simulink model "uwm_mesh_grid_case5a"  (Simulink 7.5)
settings: Solver=ode45  StartTime=0.0  StopTime=3.0  RelTol=1e-4
undefined symbols (not defined in the file or in its folder): D1, Delta, dfilt, DiscIntNeverNeededParam, Discrete, no, powergui, steady, ZData
libraries: powerlib x259, powerlib_extras x68, dsparch4 x11
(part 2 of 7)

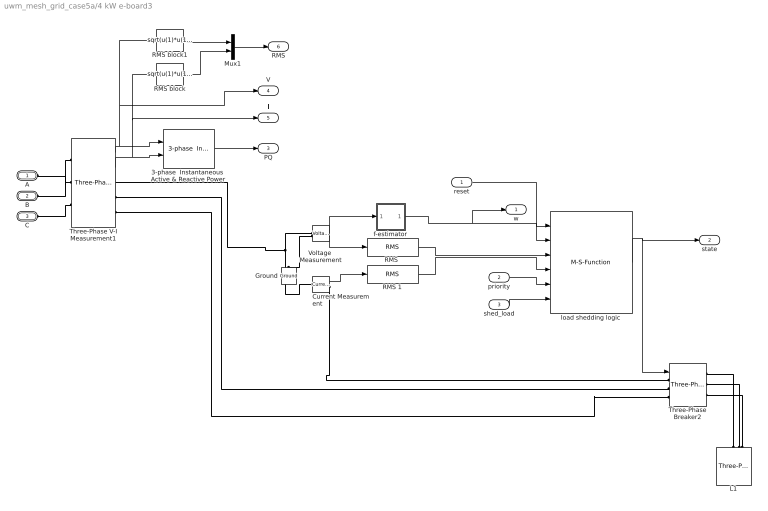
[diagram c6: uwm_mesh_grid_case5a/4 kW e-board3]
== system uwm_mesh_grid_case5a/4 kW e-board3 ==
  reset : Inport
  priority : Inport  Port=2
  shed_load : Inport  Port=3
  3-phase  Instantaneous  Active & Reactive Power : powerlib_extras/Measurements/3-phase  Instantaneous  Active & Reactive Power  DialogController=POWERSYS.PowerSysDialog  SystemSampleTime=-1
  Current Measurement : powerlib/Measurements/Current Measurement  DialogController=POWERSYS.PowerSysDialog  SystemSampleTime=-1  PhasorSimulation=off  OutputType=Complex  PSBequivalent=0
  Ground : powerlib/Elements/Ground  DialogController=POWERSYS.PowerSysDialog  PhysicalDomain=powersysdomain  SubClassName=unknown  LeftPortType=p1  RightPortType=p1  LConnTagsString=a
  L1 : powerlib/Elements/Three-Phase Series RLC Load  DialogController=POWERSYS.PowerSysDialog  PhysicalDomain=powersysdomain  SubClassName=unknown  LeftPortType=p1  RightPortType=p1  LConnTagsString=A|B|C  Configuration=Y (grounded)  NominalVoltage=208  NominalFrequency=60  ActivePower=4000  InductivePower=0  CapacitivePower=0  Measurements=None
  Mux1 : Mux  Inputs=2
  "RMS " : powerlib_extras/Measurements/RMS  DialogController=POWERSYS.PowerSysDialog  SystemSampleTime=-1  f1=60
  RMS 1 : powerlib_extras/Measurements/RMS  DialogController=POWERSYS.PowerSysDialog  SystemSampleTime=-1  f1=60
  RMS block : Fcn  Expr=sqrt(u(1)*u(1)+u(2)*u(2)+u(3)*u(3))/sqrt(3)
  RMS block1 : Fcn  Expr=sqrt(u(1)*u(1)+u(2)*u(2)+u(3)*u(3))/sqrt(3)
  Three-Phase V-I Measurement1 : powerlib/Measurements/Three-Phase V-I Measurement  DialogController=POWERSYS.PowerSysDialog  SystemSampleTime=-1  VoltageMeasurement=phase-to-ground  SetLabelV=off  LabelV=Vabc  Vpu=off  VpuLL=off  CurrentMeasurement=yes  SetLabelI=off  LabelI=Iabc  Ipu=off  Pbase=100e6  Vbase=500e3  OutputType=Complex  PhasorSimulation=off  PSBequivalent=0
  Three-Phase Breaker2 : powerlib/Elements/Three-Phase Breaker  DialogController=POWERSYS.PowerSysDialog  SystemSampleTime=-1  InitialState=closed  SwitchA=on  SwitchB=on  SwitchC=on  SwitchTimes=[50]  External=on  BreakerResistance=0.001  SnubberResistance=1e6  SnubberCapacitance=inf  Measurements=None
  Voltage  Measurement : powerlib/Measurements/Voltage Measurement  DialogController=POWERSYS.PowerSysDialog  SystemSampleTime=-1  PhasorSimulation=off  OutputType=Complex  PSBequivalent=0
  f-estimator : Subsystem  mask{dt=0.010}
      mask prompts: dt "sample time"
  load shedding logic : M-S-Function  FunctionName=load_shedding_logic3
  A : PMIOPort  Port=1  Side=Left
  B : PMIOPort  Port=2  Side=Left
  C : PMIOPort  Port=3  Side=Left
  w : Outport  OutDataType=fixdt(1, 16)  OutScaling=2^0
  state : Outport  Port=2  OutDataType=fixdt(1, 16)  OutScaling=2^0
  PQ : Outport  Port=3  OutDataType=fixdt(1, 16)  OutScaling=2^0
  V : Outport  Port=4  OutDataType=fixdt(1, 16)  OutScaling=2^0
  I : Outport  Port=5  OutDataType=fixdt(1, 16)  OutScaling=2^0
  RMS : Outport  Port=6  OutDataType=fixdt(1, 16)  OutScaling=2^0
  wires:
  reset/1 -> load shedding logic/1
  Current Measurement/1 -> RMS 1/1
  Voltage  Measurement/1 -> "RMS "/1, f-estimator/1(v)
  f-estimator/1(w) -> load shedding logic/2, w/1
  "RMS "/1 -> load shedding logic/3
  RMS 1/1 -> load shedding logic/4
  load shedding logic/1 -> Three-Phase Breaker2/1, state/1
  priority/1 -> load shedding logic/5
  Three-Phase V-I Measurement1/1 -> 3-phase  Instantaneous  Active & Reactive Power/1, RMS block1/1, V/1
  Three-Phase V-I Measurement1/2 -> 3-phase  Instantaneous  Active & Reactive Power/2, RMS block/1, I/1
  3-phase  Instantaneous  Active & Reactive Power/1 -> PQ/1
  RMS block1/1 -> Mux1/1
  RMS block/1 -> Mux1/2
  Mux1/1 -> RMS/1
  shed_load/1 -> load shedding logic/6
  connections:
  Voltage  Measurement/LConn1 -- Current Measurement/LConn1 -- Three-Phase V-I Measurement1/RConn1
  Voltage  Measurement/LConn2 -- Ground/LConn1
  Current Measurement/RConn1 -- Three-Phase Breaker2/LConn1
  L1/LConn1 -- Three-Phase Breaker2/RConn1
  L1/LConn2 -- Three-Phase Breaker2/RConn2
  L1/LConn3 -- Three-Phase Breaker2/RConn3
  Three-Phase V-I Measurement1/LConn1 -- A/RConn1
  Three-Phase V-I Measurement1/LConn2 -- B/RConn1
  Three-Phase V-I Measurement1/LConn3 -- C/RConn1
  Three-Phase V-I Measurement1/RConn2 -- Three-Phase Breaker2/LConn2
  Three-Phase V-I Measurement1/RConn3 -- Three-Phase Breaker2/LConn3

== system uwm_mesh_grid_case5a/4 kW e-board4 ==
  reset : Inport
  priority : Inport  Port=2
  shed_load : Inport  Port=3
  3-phase  Instantaneous  Active & Reactive Power : powerlib_extras/Measurements/3-phase  Instantaneous  Active & Reactive Power  DialogController=POWERSYS.PowerSysDialog  SystemSampleTime=-1
  Current Measurement : powerlib/Measurements/Current Measurement  DialogController=POWERSYS.PowerSysDialog  SystemSampleTime=-1  PhasorSimulation=off  OutputType=Complex  PSBequivalent=0
  Ground : powerlib/Elements/Ground  DialogController=POWERSYS.PowerSysDialog  PhysicalDomain=powersysdomain  SubClassName=unknown  LeftPortType=p1  RightPortType=p1  LConnTagsString=a
  L1 : powerlib/Elements/Three-Phase Series RLC Load  DialogController=POWERSYS.PowerSysDialog  PhysicalDomain=powersysdomain  SubClassName=unknown  LeftPortType=p1  RightPortType=p1  LConnTagsString=A|B|C  Configuration=Y (grounded)  NominalVoltage=208  NominalFrequency=60  ActivePower=4000  InductivePower=0  CapacitivePower=0  Measurements=None
  Mux1 : Mux  Inputs=2
  "RMS " : powerlib_extras/Measurements/RMS  DialogController=POWERSYS.PowerSysDialog  SystemSampleTime=-1  f1=60
  RMS 1 : powerlib_extras/Measurements/RMS  DialogController=POWERSYS.PowerSysDialog  SystemSampleTime=-1  f1=60
  RMS block : Fcn  Expr=sqrt(u(1)*u(1)+u(2)*u(2)+u(3)*u(3))/sqrt(3)
  RMS block1 : Fcn  Expr=sqrt(u(1)*u(1)+u(2)*u(2)+u(3)*u(3))/sqrt(3)
  Three-Phase V-I Measurement1 : powerlib/Measurements/Three-Phase V-I Measurement  DialogController=POWERSYS.PowerSysDialog  SystemSampleTime=-1  VoltageMeasurement=phase-to-ground  SetLabelV=off  LabelV=Vabc  Vpu=off  VpuLL=off  CurrentMeasurement=yes  SetLabelI=off  LabelI=Iabc  Ipu=off  Pbase=100e6  Vbase=500e3  OutputType=Complex  PhasorSimulation=off  PSBequivalent=0
  Three-Phase Breaker2 : powerlib/Elements/Three-Phase Breaker  DialogController=POWERSYS.PowerSysDialog  SystemSampleTime=-1  InitialState=closed  SwitchA=on  SwitchB=on  SwitchC=on  SwitchTimes=[50]  External=on  BreakerResistance=0.001  SnubberResistance=1e6  SnubberCapacitance=inf  Measurements=None
  Voltage  Measurement : powerlib/Measurements/Voltage Measurement  DialogController=POWERSYS.PowerSysDialog  SystemSampleTime=-1  PhasorSimulation=off  OutputType=Complex  PSBequivalent=0
  f-estimator : Subsystem  mask{dt=0.010}
      mask prompts: dt "sample time"
  load shedding logic : M-S-Function  FunctionName=load_shedding_logic3
  A : PMIOPort  Port=1  Side=Left
  B : PMIOPort  Port=2  Side=Left
  C : PMIOPort  Port=3  Side=Left
  w : Outport  OutDataType=fixdt(1, 16)  OutScaling=2^0
  state : Outport  Port=2  OutDataType=fixdt(1, 16)  OutScaling=2^0
  PQ : Outport  Port=3  OutDataType=fixdt(1, 16)  OutScaling=2^0
  V : Outport  Port=4  OutDataType=fixdt(1, 16)  OutScaling=2^0
  I : Outport  Port=5  OutDataType=fixdt(1, 16)  OutScaling=2^0
  RMS : Outport  Port=6  OutDataType=fixdt(1, 16)  OutScaling=2^0
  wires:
  reset/1 -> load shedding logic/1
  Current Measurement/1 -> RMS 1/1
  Voltage  Measurement/1 -> "RMS "/1, f-estimator/1(v)
  f-estimator/1(w) -> load shedding logic/2, w/1
  "RMS "/1 -> load shedding logic/3
  RMS 1/1 -> load shedding logic/4
  load shedding logic/1 -> Three-Phase Breaker2/1, state/1
  priority/1 -> load shedding logic/5
  Three-Phase V-I Measurement1/1 -> 3-phase  Instantaneous  Active & Reactive Power/1, RMS block1/1, V/1
  Three-Phase V-I Measurement1/2 -> 3-phase  Instantaneous  Active & Reactive Power/2, RMS block/1, I/1
  3-phase  Instantaneous  Active & Reactive Power/1 -> PQ/1
  RMS block1/1 -> Mux1/1
  RMS block/1 -> Mux1/2
  Mux1/1 -> RMS/1
  shed_load/1 -> load shedding logic/6
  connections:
  Voltage  Measurement/LConn1 -- Current Measurement/LConn1 -- Three-Phase V-I Measurement1/RConn1
  Voltage  Measurement/LConn2 -- Ground/LConn1
  Current Measurement/RConn1 -- Three-Phase Breaker2/LConn1
  L1/LConn1 -- Three-Phase Breaker2/RConn1
  L1/LConn2 -- Three-Phase Breaker2/RConn2
  L1/LConn3 -- Three-Phase Breaker2/RConn3
  Three-Phase V-I Measurement1/LConn1 -- A/RConn1
  Three-Phase V-I Measurement1/LConn2 -- B/RConn1
  Three-Phase V-I Measurement1/LConn3 -- C/RConn1
  Three-Phase V-I Measurement1/RConn2 -- Three-Phase Breaker2/LConn2
  Three-Phase V-I Measurement1/RConn3 -- Three-Phase Breaker2/LConn3

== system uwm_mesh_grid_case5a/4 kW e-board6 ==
  reset : Inport
  priority : Inport  Port=2
  shed_load : Inport  Port=3
  3-phase  Instantaneous  Active & Reactive Power : powerlib_extras/Measurements/3-phase  Instantaneous  Active & Reactive Power  DialogController=POWERSYS.PowerSysDialog  SystemSampleTime=-1
  Current Measurement : powerlib/Measurements/Current Measurement  DialogController=POWERSYS.PowerSysDialog  SystemSampleTime=-1  PhasorSimulation=off  OutputType=Complex  PSBequivalent=0
  Ground : powerlib/Elements/Ground  DialogController=POWERSYS.PowerSysDialog  PhysicalDomain=powersysdomain  SubClassName=unknown  LeftPortType=p1  RightPortType=p1  LConnTagsString=a
  L1 : powerlib/Elements/Three-Phase Series RLC Load  DialogController=POWERSYS.PowerSysDialog  PhysicalDomain=powersysdomain  SubClassName=unknown  LeftPortType=p1  RightPortType=p1  LConnTagsString=A|B|C  Configuration=Y (grounded)  NominalVoltage=208  NominalFrequency=60  ActivePower=4000  InductivePower=0  CapacitivePower=0  Measurements=None
  Mux1 : Mux  Inputs=2
  "RMS " : powerlib_extras/Measurements/RMS  DialogController=POWERSYS.PowerSysDialog  SystemSampleTime=-1  f1=60
  RMS 1 : powerlib_extras/Measurements/RMS  DialogController=POWERSYS.PowerSysDialog  SystemSampleTime=-1  f1=60
  RMS block : Fcn  Expr=sqrt(u(1)*u(1)+u(2)*u(2)+u(3)*u(3))/sqrt(3)
  RMS block1 : Fcn  Expr=sqrt(u(1)*u(1)+u(2)*u(2)+u(3)*u(3))/sqrt(3)
  Three-Phase V-I Measurement1 : powerlib/Measurements/Three-Phase V-I Measurement  DialogController=POWERSYS.PowerSysDialog  SystemSampleTime=-1  VoltageMeasurement=phase-to-ground  SetLabelV=off  LabelV=Vabc  Vpu=off  VpuLL=off  CurrentMeasurement=yes  SetLabelI=off  LabelI=Iabc  Ipu=off  Pbase=100e6  Vbase=500e3  OutputType=Complex  PhasorSimulation=off  PSBequivalent=0
  Three-Phase Breaker2 : powerlib/Elements/Three-Phase Breaker  DialogController=POWERSYS.PowerSysDialog  SystemSampleTime=-1  InitialState=closed  SwitchA=on  SwitchB=on  SwitchC=on  SwitchTimes=[50]  External=on  BreakerResistance=0.001  SnubberResistance=1e6  SnubberCapacitance=inf  Measurements=None
  Voltage  Measurement : powerlib/Measurements/Voltage Measurement  DialogController=POWERSYS.PowerSysDialog  SystemSampleTime=-1  PhasorSimulation=off  OutputType=Complex  PSBequivalent=0
  f-estimator : Subsystem  mask{dt=0.010}
      mask prompts: dt "sample time"
  load shedding logic : M-S-Function  FunctionName=load_shedding_logic3
  A : PMIOPort  Port=1  Side=Left
  B : PMIOPort  Port=2  Side=Left
  C : PMIOPort  Port=3  Side=Left
  w : Outport  OutDataType=fixdt(1, 16)  OutScaling=2^0
  state : Outport  Port=2  OutDataType=fixdt(1, 16)  OutScaling=2^0
  PQ : Outport  Port=3  OutDataType=fixdt(1, 16)  OutScaling=2^0
  V : Outport  Port=4  OutDataType=fixdt(1, 16)  OutScaling=2^0
  I : Outport  Port=5  OutDataType=fixdt(1, 16)  OutScaling=2^0
  RMS : Outport  Port=6  OutDataType=fixdt(1, 16)  OutScaling=2^0
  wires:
  reset/1 -> load shedding logic/1
  Current Measurement/1 -> RMS 1/1
  Voltage  Measurement/1 -> "RMS "/1, f-estimator/1(v)
  f-estimator/1(w) -> load shedding logic/2, w/1
  "RMS "/1 -> load shedding logic/3
  RMS 1/1 -> load shedding logic/4
  load shedding logic/1 -> Three-Phase Breaker2/1, state/1
  priority/1 -> load shedding logic/5
  Three-Phase V-I Measurement1/1 -> 3-phase  Instantaneous  Active & Reactive Power/1, RMS block1/1, V/1
  Three-Phase V-I Measurement1/2 -> 3-phase  Instantaneous  Active & Reactive Power/2, RMS block/1, I/1
  3-phase  Instantaneous  Active & Reactive Power/1 -> PQ/1
  RMS block1/1 -> Mux1/1
  RMS block/1 -> Mux1/2
  Mux1/1 -> RMS/1
  shed_load/1 -> load shedding logic/6
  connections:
  Voltage  Measurement/LConn1 -- Current Measurement/LConn1 -- Three-Phase V-I Measurement1/RConn1
  Voltage  Measurement/LConn2 -- Ground/LConn1
  Current Measurement/RConn1 -- Three-Phase Breaker2/LConn1
  L1/LConn1 -- Three-Phase Breaker2/RConn1
  L1/LConn2 -- Three-Phase Breaker2/RConn2
  L1/LConn3 -- Three-Phase Breaker2/RConn3
  Three-Phase V-I Measurement1/LConn1 -- A/RConn1
  Three-Phase V-I Measurement1/LConn2 -- B/RConn1
  Three-Phase V-I Measurement1/LConn3 -- C/RConn1
  Three-Phase V-I Measurement1/RConn2 -- Three-Phase Breaker2/LConn2
  Three-Phase V-I Measurement1/RConn3 -- Three-Phase Breaker2/LConn3

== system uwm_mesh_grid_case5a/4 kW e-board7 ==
  reset : Inport
  priority : Inport  Port=2
  shed_load : Inport  Port=3
  3-phase  Instantaneous  Active & Reactive Power : powerlib_extras/Measurements/3-phase  Instantaneous  Active & Reactive Power  DialogController=POWERSYS.PowerSysDialog  SystemSampleTime=-1
  Current Measurement : powerlib/Measurements/Current Measurement  DialogController=POWERSYS.PowerSysDialog  SystemSampleTime=-1  PhasorSimulation=off  OutputType=Complex  PSBequivalent=0
  Ground : powerlib/Elements/Ground  DialogController=POWERSYS.PowerSysDialog  PhysicalDomain=powersysdomain  SubClassName=unknown  LeftPortType=p1  RightPortType=p1  LConnTagsString=a
  L1 : powerlib/Elements/Three-Phase Series RLC Load  DialogController=POWERSYS.PowerSysDialog  PhysicalDomain=powersysdomain  SubClassName=unknown  LeftPortType=p1  RightPortType=p1  LConnTagsString=A|B|C  Configuration=Y (grounded)  NominalVoltage=208  NominalFrequency=60  ActivePower=4000  InductivePower=0  CapacitivePower=0  Measurements=None
  Mux1 : Mux  Inputs=2
  "RMS " : powerlib_extras/Measurements/RMS  DialogController=POWERSYS.PowerSysDialog  SystemSampleTime=-1  f1=60
  RMS 1 : powerlib_extras/Measurements/RMS  DialogController=POWERSYS.PowerSysDialog  SystemSampleTime=-1  f1=60
  RMS block : Fcn  Expr=sqrt(u(1)*u(1)+u(2)*u(2)+u(3)*u(3))/sqrt(3)
  RMS block1 : Fcn  Expr=sqrt(u(1)*u(1)+u(2)*u(2)+u(3)*u(3))/sqrt(3)
  Three-Phase V-I Measurement1 : powerlib/Measurements/Three-Phase V-I Measurement  DialogController=POWERSYS.PowerSysDialog  SystemSampleTime=-1  VoltageMeasurement=phase-to-ground  SetLabelV=off  LabelV=Vabc  Vpu=off  VpuLL=off  CurrentMeasurement=yes  SetLabelI=off  LabelI=Iabc  Ipu=off  Pbase=100e6  Vbase=500e3  OutputType=Complex  PhasorSimulation=off  PSBequivalent=0
  Three-Phase Breaker2 : powerlib/Elements/Three-Phase Breaker  DialogController=POWERSYS.PowerSysDialog  SystemSampleTime=-1  InitialState=closed  SwitchA=on  SwitchB=on  SwitchC=on  SwitchTimes=[50]  External=on  BreakerResistance=0.001  SnubberResistance=1e6  SnubberCapacitance=inf  Measurements=None
  Voltage  Measurement : powerlib/Measurements/Voltage Measurement  DialogController=POWERSYS.PowerSysDialog  SystemSampleTime=-1  PhasorSimulation=off  OutputType=Complex  PSBequivalent=0
  f-estimator : Subsystem  mask{dt=0.010}
      mask prompts: dt "sample time"
  load shedding logic : M-S-Function  FunctionName=load_shedding_logic3
  A : PMIOPort  Port=1  Side=Left
  B : PMIOPort  Port=2  Side=Left
  C : PMIOPort  Port=3  Side=Left
  w : Outport  OutDataType=fixdt(1, 16)  OutScaling=2^0
  state : Outport  Port=2  OutDataType=fixdt(1, 16)  OutScaling=2^0
  PQ : Outport  Port=3  OutDataType=fixdt(1, 16)  OutScaling=2^0
  V : Outport  Port=4  OutDataType=fixdt(1, 16)  OutScaling=2^0
  I : Outport  Port=5  OutDataType=fixdt(1, 16)  OutScaling=2^0
  RMS : Outport  Port=6  OutDataType=fixdt(1, 16)  OutScaling=2^0
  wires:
  reset/1 -> load shedding logic/1
  Current Measurement/1 -> RMS 1/1
  Voltage  Measurement/1 -> "RMS "/1, f-estimator/1(v)
  f-estimator/1(w) -> load shedding logic/2, w/1
  "RMS "/1 -> load shedding logic/3
  RMS 1/1 -> load shedding logic/4
  load shedding logic/1 -> Three-Phase Breaker2/1, state/1
  priority/1 -> load shedding logic/5
  Three-Phase V-I Measurement1/1 -> 3-phase  Instantaneous  Active & Reactive Power/1, RMS block1/1, V/1
  Three-Phase V-I Measurement1/2 -> 3-phase  Instantaneous  Active & Reactive Power/2, RMS block/1, I/1
  3-phase  Instantaneous  Active & Reactive Power/1 -> PQ/1
  RMS block1/1 -> Mux1/1
  RMS block/1 -> Mux1/2
  Mux1/1 -> RMS/1
  shed_load/1 -> load shedding logic/6
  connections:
  Voltage  Measurement/LConn1 -- Current Measurement/LConn1 -- Three-Phase V-I Measurement1/RConn1
  Voltage  Measurement/LConn2 -- Ground/LConn1
  Current Measurement/RConn1 -- Three-Phase Breaker2/LConn1
  L1/LConn1 -- Three-Phase Breaker2/RConn1
  L1/LConn2 -- Three-Phase Breaker2/RConn2
  L1/LConn3 -- Three-Phase Breaker2/RConn3
  Three-Phase V-I Measurement1/LConn1 -- A/RConn1
  Three-Phase V-I Measurement1/LConn2 -- B/RConn1
  Three-Phase V-I Measurement1/LConn3 -- C/RConn1
  Three-Phase V-I Measurement1/RConn2 -- Three-Phase Breaker2/LConn2
  Three-Phase V-I Measurement1/RConn3 -- Three-Phase Breaker2/LConn3

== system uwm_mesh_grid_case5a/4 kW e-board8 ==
  reset : Inport
  priority : Inport  Port=2
  shed_load : Inport  Port=3
  3-phase  Instantaneous  Active & Reactive Power : powerlib_extras/Measurements/3-phase  Instantaneous  Active & Reactive Power  DialogController=POWERSYS.PowerSysDialog  SystemSampleTime=-1
  Current Measurement : powerlib/Measurements/Current Measurement  DialogController=POWERSYS.PowerSysDialog  SystemSampleTime=-1  PhasorSimulation=off  OutputType=Complex  PSBequivalent=0
  Ground : powerlib/Elements/Ground  DialogController=POWERSYS.PowerSysDialog  PhysicalDomain=powersysdomain  SubClassName=unknown  LeftPortType=p1  RightPortType=p1  LConnTagsString=a
  L1 : powerlib/Elements/Three-Phase Series RLC Load  DialogController=POWERSYS.PowerSysDialog  PhysicalDomain=powersysdomain  SubClassName=unknown  LeftPortType=p1  RightPortType=p1  LConnTagsString=A|B|C  Configuration=Y (grounded)  NominalVoltage=208  NominalFrequency=60  ActivePower=2000  InductivePower=0  CapacitivePower=0  Measurements=None
  Mux1 : Mux  Inputs=2
  "RMS " : powerlib_extras/Measurements/RMS  DialogController=POWERSYS.PowerSysDialog  SystemSampleTime=-1  f1=60
  RMS 1 : powerlib_extras/Measurements/RMS  DialogController=POWERSYS.PowerSysDialog  SystemSampleTime=-1  f1=60
  RMS block : Fcn  Expr=sqrt(u(1)*u(1)+u(2)*u(2)+u(3)*u(3))/sqrt(3)
  RMS block1 : Fcn  Expr=sqrt(u(1)*u(1)+u(2)*u(2)+u(3)*u(3))/sqrt(3)
  Three-Phase V-I Measurement1 : powerlib/Measurements/Three-Phase V-I Measurement  DialogController=POWERSYS.PowerSysDialog  SystemSampleTime=-1  VoltageMeasurement=phase-to-ground  SetLabelV=off  LabelV=Vabc  Vpu=off  VpuLL=off  CurrentMeasurement=yes  SetLabelI=off  LabelI=Iabc  Ipu=off  Pbase=100e6  Vbase=500e3  OutputType=Complex  PhasorSimulation=off  PSBequivalent=0
  Three-Phase Breaker2 : powerlib/Elements/Three-Phase Breaker  DialogController=POWERSYS.PowerSysDialog  SystemSampleTime=-1  InitialState=closed  SwitchA=on  SwitchB=on  SwitchC=on  SwitchTimes=[50]  External=on  BreakerResistance=0.001  SnubberResistance=1e6  SnubberCapacitance=inf  Measurements=None
  Voltage  Measurement : powerlib/Measurements/Voltage Measurement  DialogController=POWERSYS.PowerSysDialog  SystemSampleTime=-1  PhasorSimulation=off  OutputType=Complex  PSBequivalent=0
  f-estimator : Subsystem  mask{dt=0.010}
      mask prompts: dt "sample time"
  load shedding logic : M-S-Function  FunctionName=load_shedding_logic3
  A : PMIOPort  Port=1  Side=Left
  B : PMIOPort  Port=2  Side=Left
  C : PMIOPort  Port=3  Side=Left
  w : Outport  OutDataType=fixdt(1, 16)  OutScaling=2^0
  state : Outport  Port=2  OutDataType=fixdt(1, 16)  OutScaling=2^0
  PQ : Outport  Port=3  OutDataType=fixdt(1, 16)  OutScaling=2^0
  V : Outport  Port=4  OutDataType=fixdt(1, 16)  OutScaling=2^0
  I : Outport  Port=5  OutDataType=fixdt(1, 16)  OutScaling=2^0
  RMS : Outport  Port=6  OutDataType=fixdt(1, 16)  OutScaling=2^0
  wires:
  reset/1 -> load shedding logic/1
  Current Measurement/1 -> RMS 1/1
  Voltage  Measurement/1 -> "RMS "/1, f-estimator/1(v)
  f-estimator/1(w) -> load shedding logic/2, w/1
  "RMS "/1 -> load shedding logic/3
  RMS 1/1 -> load shedding logic/4
  load shedding logic/1 -> Three-Phase Breaker2/1, state/1
  priority/1 -> load shedding logic/5
  Three-Phase V-I Measurement1/1 -> 3-phase  Instantaneous  Active & Reactive Power/1, RMS block1/1, V/1
  Three-Phase V-I Measurement1/2 -> 3-phase  Instantaneous  Active & Reactive Power/2, RMS block/1, I/1
  3-phase  Instantaneous  Active & Reactive Power/1 -> PQ/1
  RMS block1/1 -> Mux1/1
  RMS block/1 -> Mux1/2
  Mux1/1 -> RMS/1
  shed_load/1 -> load shedding logic/6
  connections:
  Voltage  Measurement/LConn1 -- Current Measurement/LConn1 -- Three-Phase V-I Measurement1/RConn1
  Voltage  Measurement/LConn2 -- Ground/LConn1
  Current Measurement/RConn1 -- Three-Phase Breaker2/LConn1
  L1/LConn1 -- Three-Phase Breaker2/RConn1
  L1/LConn2 -- Three-Phase Breaker2/RConn2
  L1/LConn3 -- Three-Phase Breaker2/RConn3
  Three-Phase V-I Measurement1/LConn1 -- A/RConn1
  Three-Phase V-I Measurement1/LConn2 -- B/RConn1
  Three-Phase V-I Measurement1/LConn3 -- C/RConn1
  Three-Phase V-I Measurement1/RConn2 -- Three-Phase Breaker2/LConn2
  Three-Phase V-I Measurement1/RConn3 -- Three-Phase Breaker2/LConn3

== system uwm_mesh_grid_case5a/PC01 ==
  3-phase  Instantaneous  Active & Reactive Power : powerlib_extras/Measurements/3-phase  Instantaneous  Active & Reactive Power  DialogController=POWERSYS.PowerSysDialog  SystemSampleTime=-1
  Ground : powerlib/Elements/Ground  DialogController=POWERSYS.PowerSysDialog  PhysicalDomain=powersysdomain  SubClassName=unknown  LeftPortType=p1  RightPortType=p1  LConnTagsString=a
  Three-Phase Parallel RLC Branch : powerlib/Elements/Three-Phase Parallel RLC Branch  DialogController=POWERSYS.PowerSysDialog  PhysicalDomain=powersysdomain  SubClassName=unknown  LeftPortType=p1  RightPortType=p1  LConnTagsString=A|B|C  RConnTagsString=A|B|C  BranchType=C  Resistance=1  Inductance=1e-3  Capacitance=1/(C*2*pi*60)  Measurements=None
  Three-Phase Series RLC Branch3 : powerlib/Elements/Three-Phase Series RLC Branch  DialogController=POWERSYS.PowerSysDialog  PhysicalDomain=powersysdomain  SubClassName=unknown  LeftPortType=p1  RightPortType=p1  LConnTagsString=A|B|C  RConnTagsString=A|B|C  BranchType=RL  Resistance=R  Inductance=L/(2*pi*60)  Capacitance=1/(336*2*pi*60)  Measurements=None
  Three-Phase V-I Measurement : powerlib/Measurements/Three-Phase V-I Measurement  DialogController=POWERSYS.PowerSysDialog  SystemSampleTime=-1  VoltageMeasurement=phase-to-ground  SetLabelV=off  LabelV=Vabc  Vpu=off  VpuLL=off  CurrentMeasurement=yes  SetLabelI=off  LabelI=Iabc  Ipu=off  Pbase=100e6  Vbase=500e3  OutputType=Complex  PhasorSimulation=off  PSBequivalent=0
  A* : PMIOPort  Tag=PMCPort  Port=1  Side=Right
  B* : PMIOPort  Tag=PMCPort  Port=2  Side=Right
  C* : PMIOPort  Tag=PMCPort  Port=3  Side=Right
  A : PMIOPort  Tag=PMCPort  Port=4  Side=Left
  B : PMIOPort  Tag=PMCPort  Port=5  Side=Left
  C : PMIOPort  Tag=PMCPort  Port=6  Side=Left
  PQ : Outport  OutDataType=fixdt(1, 16)  OutScaling=2^0
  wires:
  Three-Phase V-I Measurement/1 -> 3-phase  Instantaneous  Active & Reactive Power/1
  Three-Phase V-I Measurement/2 -> 3-phase  Instantaneous  Active & Reactive Power/2
  3-phase  Instantaneous  Active & Reactive Power/1 -> PQ/1
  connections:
  Three-Phase Parallel RLC Branch/LConn1 -- A*/RConn1 -- Three-Phase Series RLC Branch3/LConn1
  Three-Phase Parallel RLC Branch/LConn2 -- B*/RConn1 -- Three-Phase Series RLC Branch3/LConn2
  Three-Phase Parallel RLC Branch/LConn3 -- C*/RConn1 -- Three-Phase Series RLC Branch3/LConn3
  Ground/LConn1 -- Three-Phase Parallel RLC Branch/RConn2 -- Three-Phase Parallel RLC Branch/RConn1 -- Three-Phase Parallel RLC Branch/RConn3
  Three-Phase V-I Measurement/RConn2 -- Three-Phase Series RLC Branch3/RConn2
  Three-Phase V-I Measurement/RConn3 -- Three-Phase Series RLC Branch3/RConn3
  Three-Phase V-I Measurement/RConn1 -- Three-Phase Series RLC Branch3/RConn1
  A/RConn1 -- Three-Phase V-I Measurement/LConn1
  B/RConn1 -- Three-Phase V-I Measurement/LConn2
  C/RConn1 -- Three-Phase V-I Measurement/LConn3

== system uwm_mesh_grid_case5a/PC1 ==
  3-phase  Instantaneous  Active & Reactive Power : powerlib_extras/Measurements/3-phase  Instantaneous  Active & Reactive Power  DialogController=POWERSYS.PowerSysDialog  SystemSampleTime=-1
  Ground : powerlib/Elements/Ground  DialogController=POWERSYS.PowerSysDialog  PhysicalDomain=powersysdomain  SubClassName=unknown  LeftPortType=p1  RightPortType=p1  LConnTagsString=a
  Three-Phase Parallel RLC Branch : powerlib/Elements/Three-Phase Parallel RLC Branch  DialogController=POWERSYS.PowerSysDialog  PhysicalDomain=powersysdomain  SubClassName=unknown  LeftPortType=p1  RightPortType=p1  LConnTagsString=A|B|C  RConnTagsString=A|B|C  BranchType=C  Resistance=1  Inductance=1e-3  Capacitance=1/(C*2*pi*60)  Measurements=None
  Three-Phase Series RLC Branch3 : powerlib/Elements/Three-Phase Series RLC Branch  DialogController=POWERSYS.PowerSysDialog  PhysicalDomain=powersysdomain  SubClassName=unknown  LeftPortType=p1  RightPortType=p1  LConnTagsString=A|B|C  RConnTagsString=A|B|C  BranchType=RL  Resistance=R  Inductance=L/(2*pi*60)  Capacitance=1/(336*2*pi*60)  Measurements=None
  Three-Phase V-I Measurement : powerlib/Measurements/Three-Phase V-I Measurement  DialogController=POWERSYS.PowerSysDialog  SystemSampleTime=-1  VoltageMeasurement=phase-to-ground  SetLabelV=off  LabelV=Vabc  Vpu=off  VpuLL=off  CurrentMeasurement=yes  SetLabelI=off  LabelI=Iabc  Ipu=off  Pbase=100e6  Vbase=500e3  OutputType=Complex  PhasorSimulation=off  PSBequivalent=0
  A* : PMIOPort  Tag=PMCPort  Port=1  Side=Right
  B* : PMIOPort  Tag=PMCPort  Port=2  Side=Right
  C* : PMIOPort  Tag=PMCPort  Port=3  Side=Right
  A : PMIOPort  Tag=PMCPort  Port=4  Side=Left
  B : PMIOPort  Tag=PMCPort  Port=5  Side=Left
  C : PMIOPort  Tag=PMCPort  Port=6  Side=Left
  PQ : Outport  OutDataType=fixdt(1, 16)  OutScaling=2^0
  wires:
  Three-Phase V-I Measurement/1 -> 3-phase  Instantaneous  Active & Reactive Power/1
  Three-Phase V-I Measurement/2 -> 3-phase  Instantaneous  Active & Reactive Power/2
  3-phase  Instantaneous  Active & Reactive Power/1 -> PQ/1
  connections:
  Three-Phase Parallel RLC Branch/LConn1 -- A*/RConn1 -- Three-Phase Series RLC Branch3/LConn1
  Three-Phase Parallel RLC Branch/LConn2 -- B*/RConn1 -- Three-Phase Series RLC Branch3/LConn2
  Three-Phase Parallel RLC Branch/LConn3 -- C*/RConn1 -- Three-Phase Series RLC Branch3/LConn3
  Ground/LConn1 -- Three-Phase Parallel RLC Branch/RConn2 -- Three-Phase Parallel RLC Branch/RConn1 -- Three-Phase Parallel RLC Branch/RConn3
  Three-Phase V-I Measurement/RConn2 -- Three-Phase Series RLC Branch3/RConn2
  Three-Phase V-I Measurement/RConn3 -- Three-Phase Series RLC Branch3/RConn3
  Three-Phase V-I Measurement/RConn1 -- Three-Phase Series RLC Branch3/RConn1
  A/RConn1 -- Three-Phase V-I Measurement/LConn1
  B/RConn1 -- Three-Phase V-I Measurement/LConn2
  C/RConn1 -- Three-Phase V-I Measurement/LConn3

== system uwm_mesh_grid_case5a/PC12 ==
  3-phase  Instantaneous  Active & Reactive Power : powerlib_extras/Measurements/3-phase  Instantaneous  Active & Reactive Power  DialogController=POWERSYS.PowerSysDialog  SystemSampleTime=-1
  Ground : powerlib/Elements/Ground  DialogController=POWERSYS.PowerSysDialog  PhysicalDomain=powersysdomain  SubClassName=unknown  LeftPortType=p1  RightPortType=p1  LConnTagsString=a
  Three-Phase Parallel RLC Branch : powerlib/Elements/Three-Phase Parallel RLC Branch  DialogController=POWERSYS.PowerSysDialog  PhysicalDomain=powersysdomain  SubClassName=unknown  LeftPortType=p1  RightPortType=p1  LConnTagsString=A|B|C  RConnTagsString=A|B|C  BranchType=C  Resistance=1  Inductance=1e-3  Capacitance=1/(C*2*pi*60)  Measurements=None
  Three-Phase Series RLC Branch3 : powerlib/Elements/Three-Phase Series RLC Branch  DialogController=POWERSYS.PowerSysDialog  PhysicalDomain=powersysdomain  SubClassName=unknown  LeftPortType=p1  RightPortType=p1  LConnTagsString=A|B|C  RConnTagsString=A|B|C  BranchType=RL  Resistance=R  Inductance=L/(2*pi*60)  Capacitance=1/(336*2*pi*60)  Measurements=None
  Three-Phase V-I Measurement : powerlib/Measurements/Three-Phase V-I Measurement  DialogController=POWERSYS.PowerSysDialog  SystemSampleTime=-1  VoltageMeasurement=phase-to-ground  SetLabelV=off  LabelV=Vabc  Vpu=off  VpuLL=off  CurrentMeasurement=yes  SetLabelI=off  LabelI=Iabc  Ipu=off  Pbase=100e6  Vbase=500e3  OutputType=Complex  PhasorSimulation=off  PSBequivalent=0
  A* : PMIOPort  Tag=PMCPort  Port=1  Side=Right
  B* : PMIOPort  Tag=PMCPort  Port=2  Side=Right
  C* : PMIOPort  Tag=PMCPort  Port=3  Side=Right
  A : PMIOPort  Tag=PMCPort  Port=4  Side=Left
  B : PMIOPort  Tag=PMCPort  Port=5  Side=Left
  C : PMIOPort  Tag=PMCPort  Port=6  Side=Left
  PQ : Outport  OutDataType=fixdt(1, 16)  OutScaling=2^0
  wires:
  Three-Phase V-I Measurement/1 -> 3-phase  Instantaneous  Active & Reactive Power/1
  Three-Phase V-I Measurement/2 -> 3-phase  Instantaneous  Active & Reactive Power/2
  3-phase  Instantaneous  Active & Reactive Power/1 -> PQ/1
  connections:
  Three-Phase Parallel RLC Branch/LConn1 -- A*/RConn1 -- Three-Phase Series RLC Branch3/LConn1
  Three-Phase Parallel RLC Branch/LConn2 -- B*/RConn1 -- Three-Phase Series RLC Branch3/LConn2
  Three-Phase Parallel RLC Branch/LConn3 -- C*/RConn1 -- Three-Phase Series RLC Branch3/LConn3
  Ground/LConn1 -- Three-Phase Parallel RLC Branch/RConn2 -- Three-Phase Parallel RLC Branch/RConn1 -- Three-Phase Parallel RLC Branch/RConn3
  Three-Phase V-I Measurement/RConn2 -- Three-Phase Series RLC Branch3/RConn2
  Three-Phase V-I Measurement/RConn3 -- Three-Phase Series RLC Branch3/RConn3
  Three-Phase V-I Measurement/RConn1 -- Three-Phase Series RLC Branch3/RConn1
  A/RConn1 -- Three-Phase V-I Measurement/LConn1
  B/RConn1 -- Three-Phase V-I Measurement/LConn2
  C/RConn1 -- Three-Phase V-I Measurement/LConn3

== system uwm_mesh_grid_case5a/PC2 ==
  Ground : powerlib/Elements/Ground  DialogController=POWERSYS.PowerSysDialog  PhysicalDomain=powersysdomain  SubClassName=unknown  LeftPortType=p1  RightPortType=p1  LConnTagsString=a
  Three-Phase Parallel RLC Branch : powerlib/Elements/Three-Phase Parallel RLC Branch  DialogController=POWERSYS.PowerSysDialog  PhysicalDomain=powersysdomain  SubClassName=unknown  LeftPortType=p1  RightPortType=p1  LConnTagsString=A|B|C  RConnTagsString=A|B|C  BranchType=C  Resistance=1  Inductance=1e-3  Capacitance=1/(C*2*pi*60)  Measurements=None
  Three-Phase Series RLC Branch3 : powerlib/Elements/Three-Phase Series RLC Branch  DialogController=POWERSYS.PowerSysDialog  PhysicalDomain=powersysdomain  SubClassName=unknown  LeftPortType=p1  RightPortType=p1  LConnTagsString=A|B|C  RConnTagsString=A|B|C  BranchType=RL  Resistance=R  Inductance=L/(2*pi*60)  Capacitance=1/(336*2*pi*60)  Measurements=None
  A* : PMIOPort  Tag=PMCPort  Port=1  Side=Right
  B* : PMIOPort  Tag=PMCPort  Port=2  Side=Right
  C* : PMIOPort  Tag=PMCPort  Port=3  Side=Right
  A : PMIOPort  Tag=PMCPort  Port=4  Side=Left
  B : PMIOPort  Tag=PMCPort  Port=5  Side=Left
  C : PMIOPort  Tag=PMCPort  Port=6  Side=Left
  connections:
  Three-Phase Parallel RLC Branch/LConn1 -- A*/RConn1 -- Three-Phase Series RLC Branch3/LConn1
  Three-Phase Parallel RLC Branch/LConn2 -- B*/RConn1 -- Three-Phase Series RLC Branch3/LConn2
  Three-Phase Parallel RLC Branch/LConn3 -- C*/RConn1 -- Three-Phase Series RLC Branch3/LConn3
  Three-Phase Series RLC Branch3/RConn1 -- A/RConn1
  Three-Phase Series RLC Branch3/RConn2 -- B/RConn1
  Three-Phase Series RLC Branch3/RConn3 -- C/RConn1
  Ground/LConn1 -- Three-Phase Parallel RLC Branch/RConn2 -- Three-Phase Parallel RLC Branch/RConn3 -- Three-Phase Parallel RLC Branch/RConn1

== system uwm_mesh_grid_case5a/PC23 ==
  3-phase  Instantaneous  Active & Reactive Power : powerlib_extras/Measurements/3-phase  Instantaneous  Active & Reactive Power  DialogController=POWERSYS.PowerSysDialog  SystemSampleTime=-1
  Ground : powerlib/Elements/Ground  DialogController=POWERSYS.PowerSysDialog  PhysicalDomain=powersysdomain  SubClassName=unknown  LeftPortType=p1  RightPortType=p1  LConnTagsString=a
  Three-Phase Parallel RLC Branch : powerlib/Elements/Three-Phase Parallel RLC Branch  DialogController=POWERSYS.PowerSysDialog  PhysicalDomain=powersysdomain  SubClassName=unknown  LeftPortType=p1  RightPortType=p1  LConnTagsString=A|B|C  RConnTagsString=A|B|C  BranchType=C  Resistance=1  Inductance=1e-3  Capacitance=1/(C*2*pi*60)  Measurements=None
  Three-Phase Series RLC Branch3 : powerlib/Elements/Three-Phase Series RLC Branch  DialogController=POWERSYS.PowerSysDialog  PhysicalDomain=powersysdomain  SubClassName=unknown  LeftPortType=p1  RightPortType=p1  LConnTagsString=A|B|C  RConnTagsString=A|B|C  BranchType=RL  Resistance=R  Inductance=L/(2*pi*60)  Capacitance=1/(336*2*pi*60)  Measurements=None
  Three-Phase V-I Measurement : powerlib/Measurements/Three-Phase V-I Measurement  DialogController=POWERSYS.PowerSysDialog  SystemSampleTime=-1  VoltageMeasurement=phase-to-ground  SetLabelV=off  LabelV=Vabc  Vpu=off  VpuLL=off  CurrentMeasurement=yes  SetLabelI=off  LabelI=Iabc  Ipu=off  Pbase=100e6  Vbase=500e3  OutputType=Complex  PhasorSimulation=off  PSBequivalent=0
  A* : PMIOPort  Tag=PMCPort  Port=1  Side=Right
  B* : PMIOPort  Tag=PMCPort  Port=2  Side=Right
  C* : PMIOPort  Tag=PMCPort  Port=3  Side=Right
  A : PMIOPort  Tag=PMCPort  Port=4  Side=Left
  B : PMIOPort  Tag=PMCPort  Port=5  Side=Left
  C : PMIOPort  Tag=PMCPort  Port=6  Side=Left
  PQ : Outport  OutDataType=fixdt(1, 16)  OutScaling=2^0
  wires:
  Three-Phase V-I Measurement/1 -> 3-phase  Instantaneous  Active & Reactive Power/1
  Three-Phase V-I Measurement/2 -> 3-phase  Instantaneous  Active & Reactive Power/2
  3-phase  Instantaneous  Active & Reactive Power/1 -> PQ/1
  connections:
  Three-Phase Parallel RLC Branch/LConn1 -- A*/RConn1 -- Three-Phase Series RLC Branch3/LConn1
  Three-Phase Parallel RLC Branch/LConn2 -- B*/RConn1 -- Three-Phase Series RLC Branch3/LConn2
  Three-Phase Parallel RLC Branch/LConn3 -- C*/RConn1 -- Three-Phase Series RLC Branch3/LConn3
  Ground/LConn1 -- Three-Phase Parallel RLC Branch/RConn2 -- Three-Phase Parallel RLC Branch/RConn1 -- Three-Phase Parallel RLC Branch/RConn3
  Three-Phase V-I Measurement/RConn2 -- Three-Phase Series RLC Branch3/RConn2
  Three-Phase V-I Measurement/RConn3 -- Three-Phase Series RLC Branch3/RConn3
  Three-Phase V-I Measurement/RConn1 -- Three-Phase Series RLC Branch3/RConn1
  A/RConn1 -- Three-Phase V-I Measurement/LConn1
  B/RConn1 -- Three-Phase V-I Measurement/LConn2
  C/RConn1 -- Three-Phase V-I Measurement/LConn3

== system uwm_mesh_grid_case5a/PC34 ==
  3-phase  Instantaneous  Active & Reactive Power : powerlib_extras/Measurements/3-phase  Instantaneous  Active & Reactive Power  DialogController=POWERSYS.PowerSysDialog  SystemSampleTime=-1
  Ground : powerlib/Elements/Ground  DialogController=POWERSYS.PowerSysDialog  PhysicalDomain=powersysdomain  SubClassName=unknown  LeftPortType=p1  RightPortType=p1  LConnTagsString=a
  Three-Phase Parallel RLC Branch : powerlib/Elements/Three-Phase Parallel RLC Branch  DialogController=POWERSYS.PowerSysDialog  PhysicalDomain=powersysdomain  SubClassName=unknown  LeftPortType=p1  RightPortType=p1  LConnTagsString=A|B|C  RConnTagsString=A|B|C  BranchType=C  Resistance=1  Inductance=1e-3  Capacitance=1/(C*2*pi*60)  Measurements=None
  Three-Phase Series RLC Branch3 : powerlib/Elements/Three-Phase Series RLC Branch  DialogController=POWERSYS.PowerSysDialog  PhysicalDomain=powersysdomain  SubClassName=unknown  LeftPortType=p1  RightPortType=p1  LConnTagsString=A|B|C  RConnTagsString=A|B|C  BranchType=RL  Resistance=R  Inductance=L/(2*pi*60)  Capacitance=1/(336*2*pi*60)  Measurements=None
  Three-Phase V-I Measurement : powerlib/Measurements/Three-Phase V-I Measurement  DialogController=POWERSYS.PowerSysDialog  SystemSampleTime=-1  VoltageMeasurement=phase-to-ground  SetLabelV=off  LabelV=Vabc  Vpu=off  VpuLL=off  CurrentMeasurement=yes  SetLabelI=off  LabelI=Iabc  Ipu=off  Pbase=100e6  Vbase=500e3  OutputType=Complex  PhasorSimulation=off  PSBequivalent=0
  A* : PMIOPort  Tag=PMCPort  Port=1  Side=Right
  B* : PMIOPort  Tag=PMCPort  Port=2  Side=Right
  C* : PMIOPort  Tag=PMCPort  Port=3  Side=Right
  A : PMIOPort  Tag=PMCPort  Port=4  Side=Left
  B : PMIOPort  Tag=PMCPort  Port=5  Side=Left
  C : PMIOPort  Tag=PMCPort  Port=6  Side=Left
  PQ : Outport  OutDataType=fixdt(1, 16)  OutScaling=2^0
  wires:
  Three-Phase V-I Measurement/1 -> 3-phase  Instantaneous  Active & Reactive Power/1
  Three-Phase V-I Measurement/2 -> 3-phase  Instantaneous  Active & Reactive Power/2
  3-phase  Instantaneous  Active & Reactive Power/1 -> PQ/1
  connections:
  Three-Phase Parallel RLC Branch/LConn1 -- A*/RConn1 -- Three-Phase Series RLC Branch3/LConn1
  Three-Phase Parallel RLC Branch/LConn2 -- B*/RConn1 -- Three-Phase Series RLC Branch3/LConn2
  Three-Phase Parallel RLC Branch/LConn3 -- C*/RConn1 -- Three-Phase Series RLC Branch3/LConn3
  Ground/LConn1 -- Three-Phase Parallel RLC Branch/RConn2 -- Three-Phase Parallel RLC Branch/RConn1 -- Three-Phase Parallel RLC Branch/RConn3
  Three-Phase V-I Measurement/RConn2 -- Three-Phase Series RLC Branch3/RConn2
  Three-Phase V-I Measurement/RConn3 -- Three-Phase Series RLC Branch3/RConn3
  Three-Phase V-I Measurement/RConn1 -- Three-Phase Series RLC Branch3/RConn1
  A/RConn1 -- Three-Phase V-I Measurement/LConn1
  B/RConn1 -- Three-Phase V-I Measurement/LConn2
  C/RConn1 -- Three-Phase V-I Measurement/LConn3

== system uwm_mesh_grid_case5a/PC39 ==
  3-phase  Instantaneous  Active & Reactive Power : powerlib_extras/Measurements/3-phase  Instantaneous  Active & Reactive Power  DialogController=POWERSYS.PowerSysDialog  SystemSampleTime=-1
  Ground : powerlib/Elements/Ground  DialogController=POWERSYS.PowerSysDialog  PhysicalDomain=powersysdomain  SubClassName=unknown  LeftPortType=p1  RightPortType=p1  LConnTagsString=a
  Three-Phase Parallel RLC Branch : powerlib/Elements/Three-Phase Parallel RLC Branch  DialogController=POWERSYS.PowerSysDialog  PhysicalDomain=powersysdomain  SubClassName=unknown  LeftPortType=p1  RightPortType=p1  LConnTagsString=A|B|C  RConnTagsString=A|B|C  BranchType=C  Resistance=1  Inductance=1e-3  Capacitance=1/(C*2*pi*60)  Measurements=None
  Three-Phase Series RLC Branch3 : powerlib/Elements/Three-Phase Series RLC Branch  DialogController=POWERSYS.PowerSysDialog  PhysicalDomain=powersysdomain  SubClassName=unknown  LeftPortType=p1  RightPortType=p1  LConnTagsString=A|B|C  RConnTagsString=A|B|C  BranchType=RL  Resistance=R  Inductance=L/(2*pi*60)  Capacitance=1/(336*2*pi*60)  Measurements=None
  Three-Phase V-I Measurement : powerlib/Measurements/Three-Phase V-I Measurement  DialogController=POWERSYS.PowerSysDialog  SystemSampleTime=-1  VoltageMeasurement=phase-to-ground  SetLabelV=off  LabelV=Vabc  Vpu=off  VpuLL=off  CurrentMeasurement=yes  SetLabelI=off  LabelI=Iabc  Ipu=off  Pbase=100e6  Vbase=500e3  OutputType=Complex  PhasorSimulation=off  PSBequivalent=0
  A* : PMIOPort  Tag=PMCPort  Port=1  Side=Right
  B* : PMIOPort  Tag=PMCPort  Port=2  Side=Right
  C* : PMIOPort  Tag=PMCPort  Port=3  Side=Right
  A : PMIOPort  Tag=PMCPort  Port=4  Side=Left
  B : PMIOPort  Tag=PMCPort  Port=5  Side=Left
  C : PMIOPort  Tag=PMCPort  Port=6  Side=Left
  PQ : Outport  OutDataType=fixdt(1, 16)  OutScaling=2^0
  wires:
  Three-Phase V-I Measurement/1 -> 3-phase  Instantaneous  Active & Reactive Power/1
  Three-Phase V-I Measurement/2 -> 3-phase  Instantaneous  Active & Reactive Power/2
  3-phase  Instantaneous  Active & Reactive Power/1 -> PQ/1
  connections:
  Three-Phase Parallel RLC Branch/LConn1 -- A*/RConn1 -- Three-Phase Series RLC Branch3/LConn1
  Three-Phase Parallel RLC Branch/LConn2 -- B*/RConn1 -- Three-Phase Series RLC Branch3/LConn2
  Three-Phase Parallel RLC Branch/LConn3 -- C*/RConn1 -- Three-Phase Series RLC Branch3/LConn3
  Ground/LConn1 -- Three-Phase Parallel RLC Branch/RConn2 -- Three-Phase Parallel RLC Branch/RConn1 -- Three-Phase Parallel RLC Branch/RConn3
  Three-Phase V-I Measurement/RConn2 -- Three-Phase Series RLC Branch3/RConn2
  Three-Phase V-I Measurement/RConn3 -- Three-Phase Series RLC Branch3/RConn3
  Three-Phase V-I Measurement/RConn1 -- Three-Phase Series RLC Branch3/RConn1
  A/RConn1 -- Three-Phase V-I Measurement/LConn1
  B/RConn1 -- Three-Phase V-I Measurement/LConn2
  C/RConn1 -- Three-Phase V-I Measurement/LConn3

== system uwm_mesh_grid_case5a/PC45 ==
  3-phase  Instantaneous  Active & Reactive Power : powerlib_extras/Measurements/3-phase  Instantaneous  Active & Reactive Power  DialogController=POWERSYS.PowerSysDialog  SystemSampleTime=-1
  Ground : powerlib/Elements/Ground  DialogController=POWERSYS.PowerSysDialog  PhysicalDomain=powersysdomain  SubClassName=unknown  LeftPortType=p1  RightPortType=p1  LConnTagsString=a
  Three-Phase Parallel RLC Branch : powerlib/Elements/Three-Phase Parallel RLC Branch  DialogController=POWERSYS.PowerSysDialog  PhysicalDomain=powersysdomain  SubClassName=unknown  LeftPortType=p1  RightPortType=p1  LConnTagsString=A|B|C  RConnTagsString=A|B|C  BranchType=C  Resistance=1  Inductance=1e-3  Capacitance=1/(C*2*pi*60)  Measurements=None
  Three-Phase Series RLC Branch3 : powerlib/Elements/Three-Phase Series RLC Branch  DialogController=POWERSYS.PowerSysDialog  PhysicalDomain=powersysdomain  SubClassName=unknown  LeftPortType=p1  RightPortType=p1  LConnTagsString=A|B|C  RConnTagsString=A|B|C  BranchType=RL  Resistance=R  Inductance=L/(2*pi*60)  Capacitance=1/(336*2*pi*60)  Measurements=None
  Three-Phase V-I Measurement : powerlib/Measurements/Three-Phase V-I Measurement  DialogController=POWERSYS.PowerSysDialog  SystemSampleTime=-1  VoltageMeasurement=phase-to-ground  SetLabelV=off  LabelV=Vabc  Vpu=off  VpuLL=off  CurrentMeasurement=yes  SetLabelI=off  LabelI=Iabc  Ipu=off  Pbase=100e6  Vbase=500e3  OutputType=Complex  PhasorSimulation=off  PSBequivalent=0
  A* : PMIOPort  Tag=PMCPort  Port=1  Side=Right
  B* : PMIOPort  Tag=PMCPort  Port=2  Side=Right
  C* : PMIOPort  Tag=PMCPort  Port=3  Side=Right
  A : PMIOPort  Tag=PMCPort  Port=4  Side=Left
  B : PMIOPort  Tag=PMCPort  Port=5  Side=Left
  C : PMIOPort  Tag=PMCPort  Port=6  Side=Left
  PQ : Outport  OutDataType=fixdt(1, 16)  OutScaling=2^0
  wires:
  Three-Phase V-I Measurement/1 -> 3-phase  Instantaneous  Active & Reactive Power/1
  Three-Phase V-I Measurement/2 -> 3-phase  Instantaneous  Active & Reactive Power/2
  3-phase  Instantaneous  Active & Reactive Power/1 -> PQ/1
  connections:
  Three-Phase Parallel RLC Branch/LConn1 -- A*/RConn1 -- Three-Phase Series RLC Branch3/LConn1
  Three-Phase Parallel RLC Branch/LConn2 -- B*/RConn1 -- Three-Phase Series RLC Branch3/LConn2
  Three-Phase Parallel RLC Branch/LConn3 -- C*/RConn1 -- Three-Phase Series RLC Branch3/LConn3
  Ground/LConn1 -- Three-Phase Parallel RLC Branch/RConn2 -- Three-Phase Parallel RLC Branch/RConn1 -- Three-Phase Parallel RLC Branch/RConn3
  Three-Phase V-I Measurement/RConn2 -- Three-Phase Series RLC Branch3/RConn2
  Three-Phase V-I Measurement/RConn3 -- Three-Phase Series RLC Branch3/RConn3
  Three-Phase V-I Measurement/RConn1 -- Three-Phase Series RLC Branch3/RConn1
  A/RConn1 -- Three-Phase V-I Measurement/LConn1
  B/RConn1 -- Three-Phase V-I Measurement/LConn2
  C/RConn1 -- Three-Phase V-I Measurement/LConn3

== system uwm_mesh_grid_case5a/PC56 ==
  3-phase  Instantaneous  Active & Reactive Power : powerlib_extras/Measurements/3-phase  Instantaneous  Active & Reactive Power  DialogController=POWERSYS.PowerSysDialog  SystemSampleTime=-1
  Ground : powerlib/Elements/Ground  DialogController=POWERSYS.PowerSysDialog  PhysicalDomain=powersysdomain  SubClassName=unknown  LeftPortType=p1  RightPortType=p1  LConnTagsString=a
  Three-Phase Parallel RLC Branch : powerlib/Elements/Three-Phase Parallel RLC Branch  DialogController=POWERSYS.PowerSysDialog  PhysicalDomain=powersysdomain  SubClassName=unknown  LeftPortType=p1  RightPortType=p1  LConnTagsString=A|B|C  RConnTagsString=A|B|C  BranchType=C  Resistance=1  Inductance=1e-3  Capacitance=1/(C*2*pi*60)  Measurements=None
  Three-Phase Series RLC Branch3 : powerlib/Elements/Three-Phase Series RLC Branch  DialogController=POWERSYS.PowerSysDialog  PhysicalDomain=powersysdomain  SubClassName=unknown  LeftPortType=p1  RightPortType=p1  LConnTagsString=A|B|C  RConnTagsString=A|B|C  BranchType=RL  Resistance=R  Inductance=L/(2*pi*60)  Capacitance=1/(336*2*pi*60)  Measurements=None
  Three-Phase V-I Measurement : powerlib/Measurements/Three-Phase V-I Measurement  DialogController=POWERSYS.PowerSysDialog  SystemSampleTime=-1  VoltageMeasurement=phase-to-ground  SetLabelV=off  LabelV=Vabc  Vpu=off  VpuLL=off  CurrentMeasurement=yes  SetLabelI=off  LabelI=Iabc  Ipu=off  Pbase=100e6  Vbase=500e3  OutputType=Complex  PhasorSimulation=off  PSBequivalent=0
  A* : PMIOPort  Tag=PMCPort  Port=1  Side=Right
  B* : PMIOPort  Tag=PMCPort  Port=2  Side=Right
  C* : PMIOPort  Tag=PMCPort  Port=3  Side=Right
  A : PMIOPort  Tag=PMCPort  Port=4  Side=Left
  B : PMIOPort  Tag=PMCPort  Port=5  Side=Left
  C : PMIOPort  Tag=PMCPort  Port=6  Side=Left
  PQ : Outport  OutDataType=fixdt(1, 16)  OutScaling=2^0
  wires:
  Three-Phase V-I Measurement/1 -> 3-phase  Instantaneous  Active & Reactive Power/1
  Three-Phase V-I Measurement/2 -> 3-phase  Instantaneous  Active & Reactive Power/2
  3-phase  Instantaneous  Active & Reactive Power/1 -> PQ/1
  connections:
  Three-Phase Parallel RLC Branch/LConn1 -- A*/RConn1 -- Three-Phase Series RLC Branch3/LConn1
  Three-Phase Parallel RLC Branch/LConn2 -- B*/RConn1 -- Three-Phase Series RLC Branch3/LConn2
  Three-Phase Parallel RLC Branch/LConn3 -- C*/RConn1 -- Three-Phase Series RLC Branch3/LConn3
  Ground/LConn1 -- Three-Phase Parallel RLC Branch/RConn2 -- Three-Phase Parallel RLC Branch/RConn1 -- Three-Phase Parallel RLC Branch/RConn3
  Three-Phase V-I Measurement/RConn2 -- Three-Phase Series RLC Branch3/RConn2
  Three-Phase V-I Measurement/RConn3 -- Three-Phase Series RLC Branch3/RConn3
  Three-Phase V-I Measurement/RConn1 -- Three-Phase Series RLC Branch3/RConn1
  A/RConn1 -- Three-Phase V-I Measurement/LConn1
  B/RConn1 -- Three-Phase V-I Measurement/LConn2
  C/RConn1 -- Three-Phase V-I Measurement/LConn3

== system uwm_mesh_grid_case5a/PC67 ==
  3-phase  Instantaneous  Active & Reactive Power : powerlib_extras/Measurements/3-phase  Instantaneous  Active & Reactive Power  DialogController=POWERSYS.PowerSysDialog  SystemSampleTime=-1
  Ground : powerlib/Elements/Ground  DialogController=POWERSYS.PowerSysDialog  PhysicalDomain=powersysdomain  SubClassName=unknown  LeftPortType=p1  RightPortType=p1  LConnTagsString=a
  Three-Phase Parallel RLC Branch : powerlib/Elements/Three-Phase Parallel RLC Branch  DialogController=POWERSYS.PowerSysDialog  PhysicalDomain=powersysdomain  SubClassName=unknown  LeftPortType=p1  RightPortType=p1  LConnTagsString=A|B|C  RConnTagsString=A|B|C  BranchType=C  Resistance=1  Inductance=1e-3  Capacitance=1/(C*2*pi*60)  Measurements=None
  Three-Phase Series RLC Branch3 : powerlib/Elements/Three-Phase Series RLC Branch  DialogController=POWERSYS.PowerSysDialog  PhysicalDomain=powersysdomain  SubClassName=unknown  LeftPortType=p1  RightPortType=p1  LConnTagsString=A|B|C  RConnTagsString=A|B|C  BranchType=RL  Resistance=R  Inductance=L/(2*pi*60)  Capacitance=1/(336*2*pi*60)  Measurements=None
  Three-Phase V-I Measurement : powerlib/Measurements/Three-Phase V-I Measurement  DialogController=POWERSYS.PowerSysDialog  SystemSampleTime=-1  VoltageMeasurement=phase-to-ground  SetLabelV=off  LabelV=Vabc  Vpu=off  VpuLL=off  CurrentMeasurement=yes  SetLabelI=off  LabelI=Iabc  Ipu=off  Pbase=100e6  Vbase=500e3  OutputType=Complex  PhasorSimulation=off  PSBequivalent=0
  A* : PMIOPort  Tag=PMCPort  Port=1  Side=Right
  B* : PMIOPort  Tag=PMCPort  Port=2  Side=Right
  C* : PMIOPort  Tag=PMCPort  Port=3  Side=Right
  A : PMIOPort  Tag=PMCPort  Port=4  Side=Left
  B : PMIOPort  Tag=PMCPort  Port=5  Side=Left
  C : PMIOPort  Tag=PMCPort  Port=6  Side=Left
  PQ : Outport  OutDataType=fixdt(1, 16)  OutScaling=2^0
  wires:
  Three-Phase V-I Measurement/1 -> 3-phase  Instantaneous  Active & Reactive Power/1
  Three-Phase V-I Measurement/2 -> 3-phase  Instantaneous  Active & Reactive Power/2
  3-phase  Instantaneous  Active & Reactive Power/1 -> PQ/1
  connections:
  Three-Phase Parallel RLC Branch/LConn1 -- A*/RConn1 -- Three-Phase Series RLC Branch3/LConn1
  Three-Phase Parallel RLC Branch/LConn2 -- B*/RConn1 -- Three-Phase Series RLC Branch3/LConn2
  Three-Phase Parallel RLC Branch/LConn3 -- C*/RConn1 -- Three-Phase Series RLC Branch3/LConn3
  Ground/LConn1 -- Three-Phase Parallel RLC Branch/RConn2 -- Three-Phase Parallel RLC Branch/RConn1 -- Three-Phase Parallel RLC Branch/RConn3
  Three-Phase V-I Measurement/RConn2 -- Three-Phase Series RLC Branch3/RConn2
  Three-Phase V-I Measurement/RConn3 -- Three-Phase Series RLC Branch3/RConn3
  Three-Phase V-I Measurement/RConn1 -- Three-Phase Series RLC Branch3/RConn1
  A/RConn1 -- Three-Phase V-I Measurement/LConn1
  B/RConn1 -- Three-Phase V-I Measurement/LConn2
  C/RConn1 -- Three-Phase V-I Measurement/LConn3
